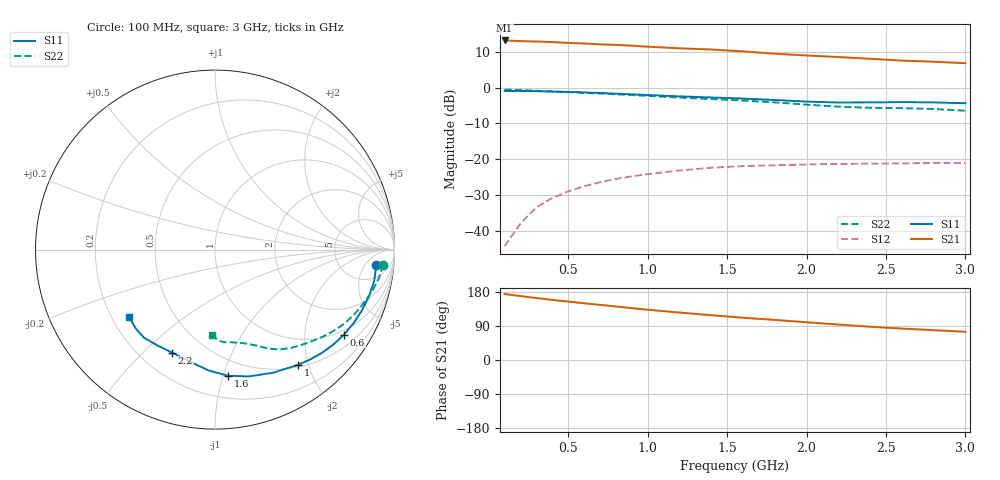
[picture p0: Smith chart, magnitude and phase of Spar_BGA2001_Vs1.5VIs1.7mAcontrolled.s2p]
! Filename: 1_51_7G1.001
! Title: BGA2001 X0297-20 HFE=80
! Bias: Vce=1.5V; Ic=1.7mA controlled / noise data included
! Company: NXP Semiconductors NL
! User: Quality&Reliability T&D
! Measure time: 23 Oct 1998 / 08:33:22
#  MHz  S  MA  R 50
! Freq  S11  S21  S12  S22  :
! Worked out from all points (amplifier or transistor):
!   20 points, 100 MHz to 3 GHz, reference 50 ohm
!   highest |S21| = 13.3 dB at 100 MHz (marker M1)
!   |S21| within 3 dB of that: start of sweep to 1.576 GHz
!   unconditionally stable (mu >= 1): 2.905 GHz to end of sweep
!   at 400 MHz: K = 0.17, MSG = 21.8 dB, |S12| = -30.9 dB
!   at 1.2 GHz: K = 0.36, MSG = 17.1 dB, |S12| = -23.2 dB
!   at 3 GHz: K = 1.07, MAG = 12.4 dB, |S12| = -21.1 dB
!   lowest NFmin = 1.10 dB at 1.8 GHz
!   S11 on the Smith chart (normalised r, x): 100 MHz: 11, -10; 600 MHz: 0.85, -3.12; 1 GHz: 0.53, -1.83; 1.6 GHz: 0.37, -1.04; 2.2 GHz: 0.33, -0.62; 3 GHz: 0.27, -0.33
100  0.9031 -5.4  4.599 174.1  0.006056 57.4  0.9399 -5.1
200  0.9041 -11.1  4.5 168.7  0.0126 82.9  0.9267 -9.9
300  0.8965 -16.9  4.447 163.5  0.02126 80.0  0.9077 -14.4
400  0.8859 -22.6  4.367 158.7  0.02866 75.9  0.8868 -18.4
500  0.8742 -28.0  4.249 154.2  0.03546 72.2  0.8694 -22.2
600  0.8606 -33.4  4.171 149.8  0.04179 68.8  0.8503 -25.9
700  0.8459 -38.6  4.058 145.5  0.04753 65.6  0.8329 -29.3
800  0.8282 -44.0  3.99 141.2  0.05293 62.5  0.8119 -32.7
900  0.8095 -49.2  3.887 136.7  0.05756 59.5  0.7912 -36.0
1000  0.791 -54.3  3.76 132.8  0.06175 56.9  0.7702 -39.3
1200  0.7583 -64.8  3.57 125.2  0.06944 51.9  0.7292 -45.7
1400  0.7315 -75.1  3.439 118.2  0.07599 47.4  0.695 -51.9
1600  0.7059 -84.2  3.232 111.5  0.08 44.0  0.6626 -57.2
1800  0.6747 -92.9  2.998 105.8  0.08219 41.8  0.6249 -61.8
2000  0.6408 -102.3  2.835 99.6  0.08428 38.8  0.5807 -66.9
2200  0.6218 -112.6  2.694 93.6  0.08586 35.8  0.5443 -73.1
2400  0.6233 -121.7  2.547 87.8  0.08677 34.1  0.525 -79.7
2600  0.6305 -128.8  2.402 82.9  0.08721 34.1  0.5183 -84.7
2800  0.6234 -135.0  2.318 78.7  0.08857 33.2  0.5047 -88.1
3000  0.608 -141.6  2.21 74.5  0.0886 33.3  0.4776 -91.8
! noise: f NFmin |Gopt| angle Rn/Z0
900  1.15  0.51  20.7  0.4
1000  1.22  0.5  21.6  0.39
1800  1.096  0.449  67.3  0.326
2000  1.197  0.425  76.26  0.289
2200  1.453  0.366  86.76  0.257
2400  1.622  0.356  99.07  0.244
